PROGRAM MAIN
VAR
	ST_Novram1: DUT_Novram_Struct;
END_VAR

VAR RETAIN
	b_bool: BOOL;
	i_int: INT;
	f_real: REAL;
	arr_Array: ARRAY[0..1023] OF byte;
	ST_Novram2: DUT_GVL_Novram_Struct;
END_VAR

END_PROGRAM
